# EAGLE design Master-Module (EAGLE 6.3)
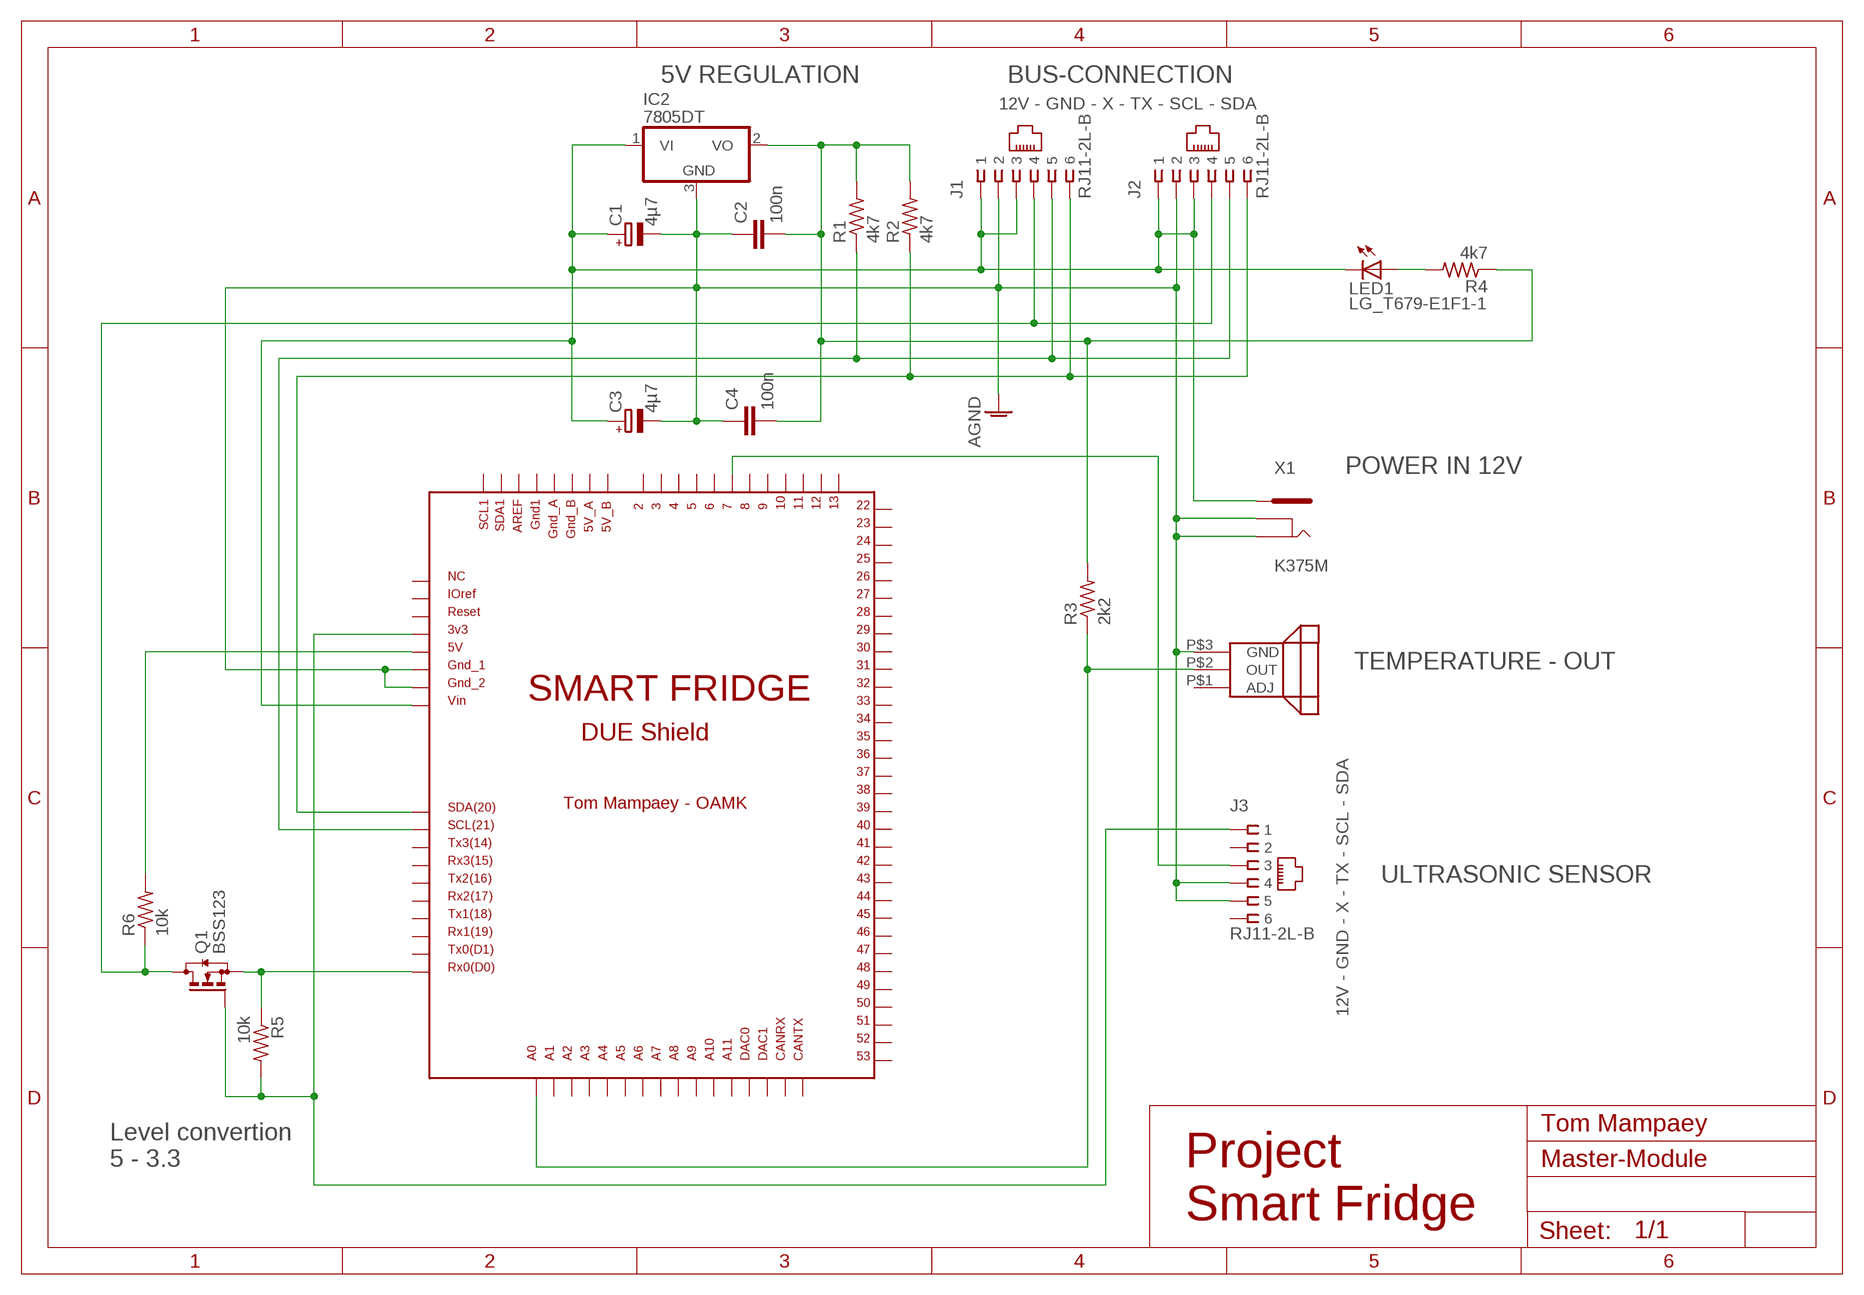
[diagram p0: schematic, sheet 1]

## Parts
C1  4µ7  CPOL-EUB  [PANASONIC_B]
C2  100n  C-EUC0603  [C0603]
C3  4µ7  CPOL-EUB  [PANASONIC_B]
C4  100n  C-EUC0603  [C0603]
IC2  7805DT  [TO252]
J1  RJ11-2L-B  [RJ11-NO_SHIELD]
J2  RJ11-2L-B  [RJ11-NO_SHIELD]
J3  RJ11-2L-B  [RJ11-NO_SHIELD]
LED1  LG_T679-E1F1-1  [PLCC2]
Q1  BSS123  [SOT23]
R1  4k7  R-US_R0402  [R0402]
R2  4k7  R-US_R0402  [R0402]
R3  2k2  R-US_R0402  [R0402]
R4  4k7  R-US_R0402  [R0402]
R5  10k  R-US_R0402  [R0402]
R6  10k  R-US_R0402  [R0402]
U$1  DUE(NORMAL)  [DUE(NORMAL)]
U$2  LM335  [LM335]
X1  K375M  [K375M]

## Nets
AGND: C1.- C2.1 C3.- C4.1 IC2.3(GND) J1.2 J2.2 J3.4 J3.5 U$1.GND_1 U$1.GND_2 U$2.P$3(GND) X1.P$1 X1.P$6
N$1: J1.6 J2.6 R2.1 U$1.SDA
N$2: J1.4 J2.4 Q1.3(D) R6.1
N$3: J1.5 J2.5 R1.1 U$1.SCL
N$4: R6.2 U$1.5V
N$5: R3.1 U$1.A0 U$2.P$2(OUT)
N$6: J3.3 U$1.7
N$7: LED1.A R4.2
N$8: C2.2 C4.2 IC2.2(VO) R1.2 R2.2 R3.2 R4.1
N$9: Q1.2(S) R5.1 U$1.RX0
N$10: C1.+ C3.+ IC2.1(VI) J1.1 J1.3 J2.1 J2.3 LED1.C U$1.VIN X1.P$7
N$14: J3.1 Q1.1(G) R5.2 U$1.3V3
Unconnected: J3.2 J3.6 U$1.2 U$1.3 U$1.4 U$1.5 U$1.5V_A U$1.5V_B U$1.6 U$1.8 U$1.9 U$1.10 U$1.11 U$1.12 U$1.13 U$1.22 U$1.23 U$1.24 U$1.25 U$1.26 U$1.27 U$1.28 U$1.29 U$1.30 U$1.31 U$1.32 U$1.33 U$1.34 U$1.35 U$1.36 U$1.37 U$1.38 U$1.39 U$1.40 U$1.41 U$1.42 U$1.43 U$1.44 U$1.45 U$1.46 U$1.47 U$1.48 U$1.49 U$1.50 U$1.51 U$1.52 U$1.53 U$1.A1 U$1.A2 U$1.A3 U$1.A4 U$1.A5 U$1.A6 U$1.A7 U$1.A8 U$1.A9 U$1.A10 U$1.A11 U$1.AREF U$1.CANRX U$1.CANTX U$1.DAC0 U$1.DAC1 U$1.GND1 U$1.GND_A U$1.GND_B U$1.IOREF U$1.NC U$1.RESET U$1.RX1 U$1.RX2 U$1.RX3 U$1.SCL1 U$1.SDA1 U$1.TX0 U$1.TX1 U$1.TX2 U$1.TX3 U$2.P$1(ADJ)

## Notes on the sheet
- 5V REGULATION | BUS-CONNECTION
- 12V - GND - X - TX - SCL - SDA
- POWER IN 12V
- TEMPERATURE - OUT
- 12V - GND - X - TX - SCL - SDA
- ULTRASONIC SENSOR
- Tom Mampaey
- Level convertion
  5 - 3.3
- Project 
  Smart Fridge

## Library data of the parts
C1 C3 = resistor:CPOL-EU: POLARIZED CAPACITOR, European symbol
C2 C4 = resistor:C-EU: CAPACITOR, European symbol
IC2 = linear:78*: Positive VOLTAGE REGULATOR Source: http://cache.national.com/ds/LM/LM78L05.pdf http://www.fairchildsemi.com/ds/LM/LM7805.pdf
J1-J3 = con-tycoelectronics:RJ11: CORCOM Modular RJ Jacks No Shield Source: www.tycoelectronics.com .. ENG_DS_1654001_1099_RJ_L_0507.pdf; MF: TYCO ELECTRONICS; MPN: RJ11-2L-B; OC_FARNELL: unknown; OC_NEWARK: 83F4463
LED1 = led:*_T679-?-1: LC TOPLED® Low Current LED; COLOR: green
Q1 = transistor-small-signal:BSS123: N-CHANNEL MOS FET
R1-R6 = rcl:R-US_: RESISTOR, American symbol
U$1 = DUE-shield custom:DUE(NORMAL)
U$2 = LM335:LM335
X1 = con-power c:K375M: K375M - DC POWER JACK 2.5mm/CENTRAL PIN Source: Data sheet

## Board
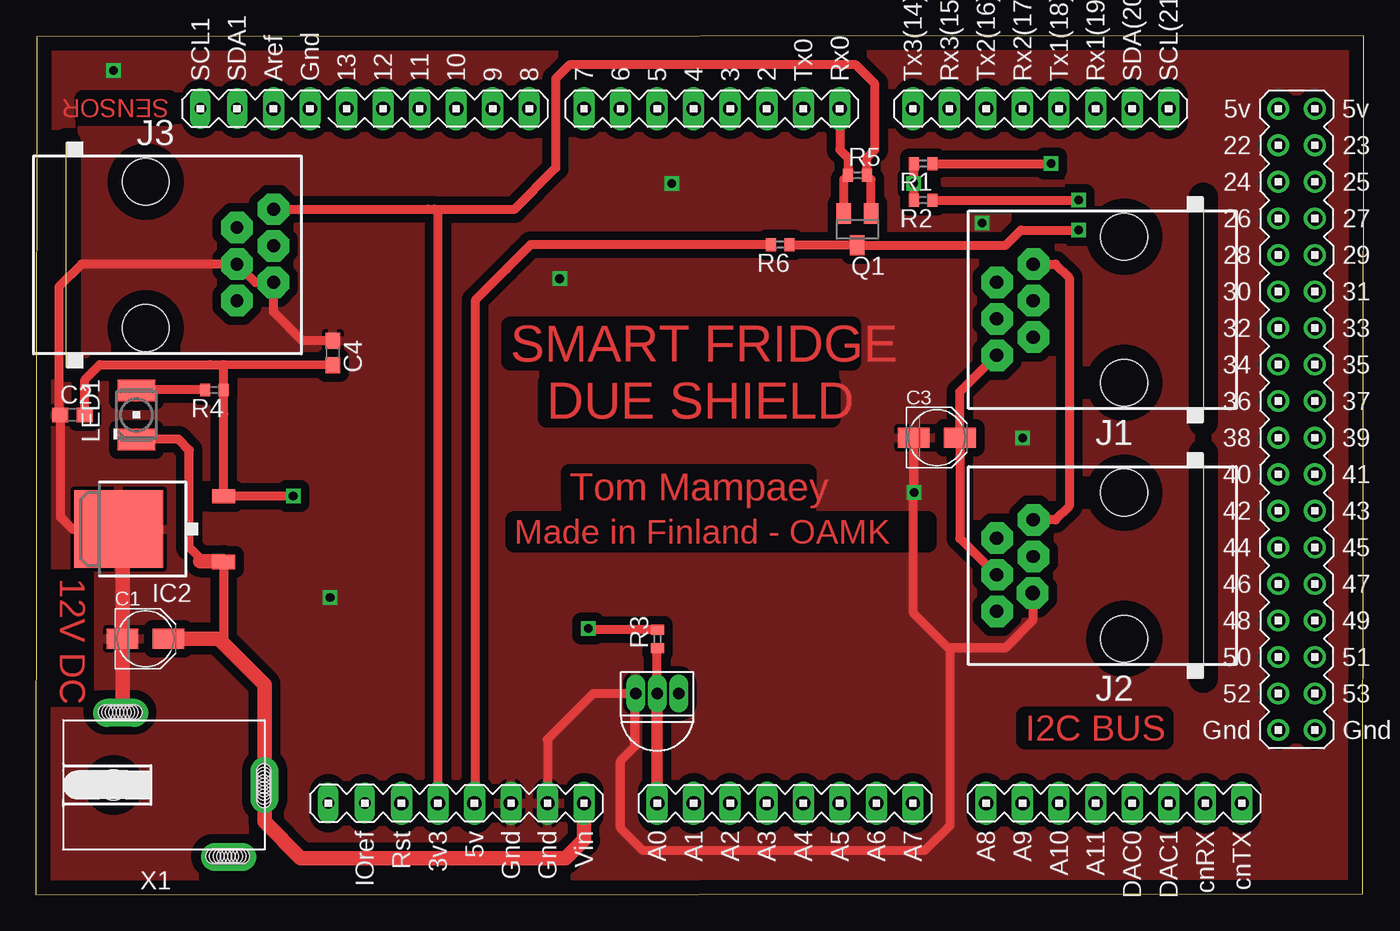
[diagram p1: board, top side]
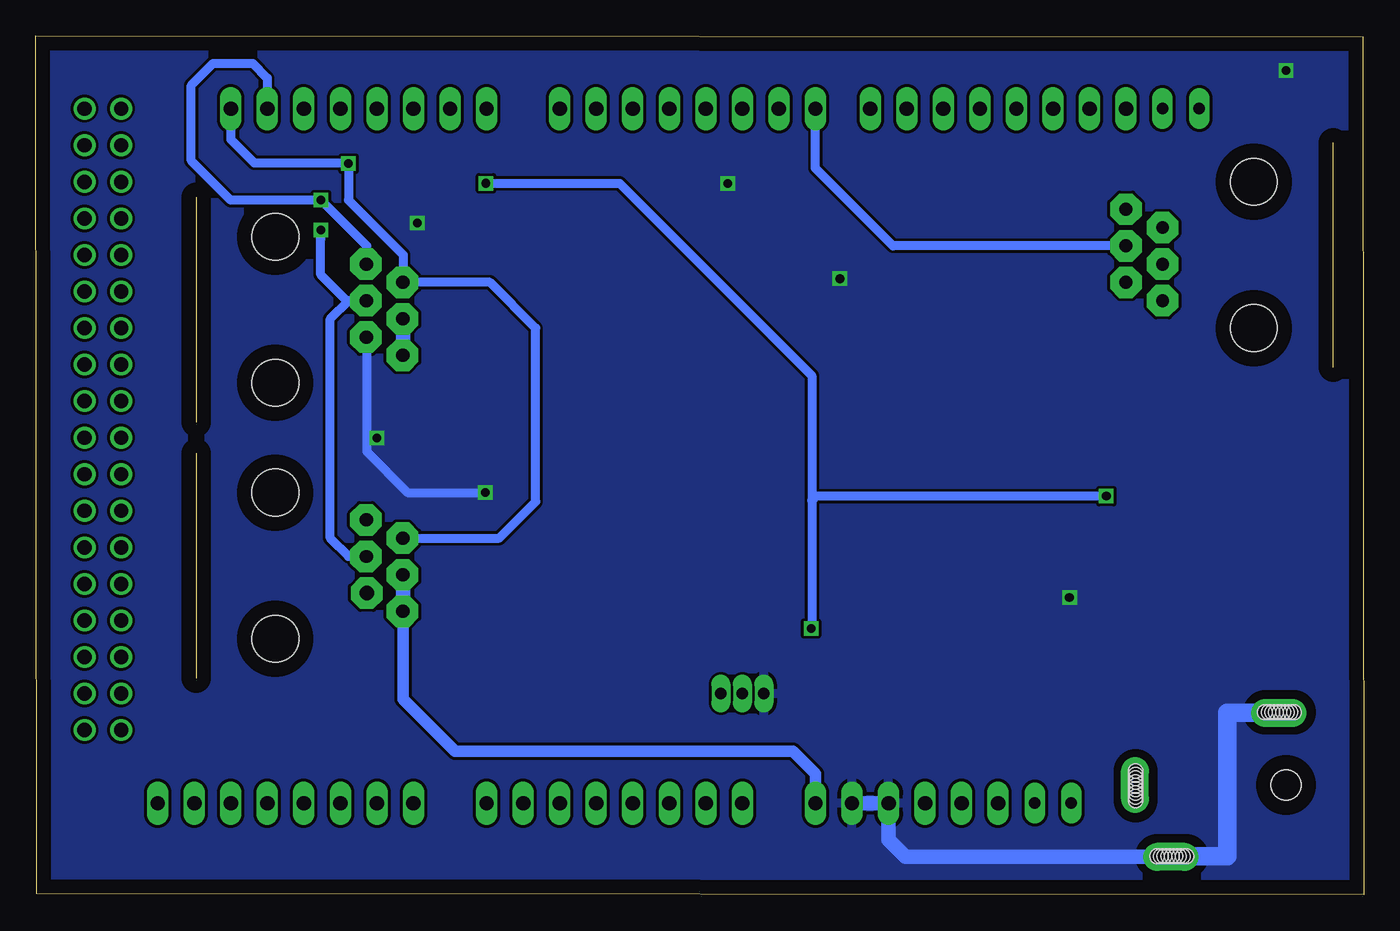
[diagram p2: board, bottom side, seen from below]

Size 92.28 x 59.66 mm. Coordinates in mm from the lower left corner, seen from the top.
Outline: 0,0 92.23,0.05 92.28,59.66 0.05,59.61 0,0
Copper layers (1*16): Top 0.035mm / dielectric 1.5mm / Bottom 0.035mm
Design rules "default": minimum track width 10mil, minimum drill 24mil, track to track 8mil, track to pad 8mil, pad to pad 8mil, via to via 8mil, smd to smd 8mil, copper to edge 40mil, drill to drill 8mil, minimum pad ring 10mil, minimum via ring 8mil, stop-mask expansion 4mil, vias tented up to drill 0mil, thermal gap 10mil

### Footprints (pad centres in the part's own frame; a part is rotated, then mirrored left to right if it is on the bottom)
PANASONIC_B = smd 2.2 x 1.4: + 1.6,0; - -1.6,0
C0603 = smd 1.1 x 1: 1 -0.85,0; 2 0.85,0
TO252 = smd 1 x 1.6: 1 -2.28,-4.8; 2 2.28,-4.8 | smd 5.4 x 6.2: 3 0,2.5
RJ11-NO_SHIELD = drill 0.9 pad 1.4: 1 -3.175,8.89; 2 -1.905,6.35; 3 -0.635,8.89; 4 0.635,6.35; 5 1.905,8.89; 6 3.175,6.35 | hole 3.251: -5.08,0; 5.08,0
PLCC2 = smd 2.6 x 1.5: A 0,1.7; C 0,-1.7
SOT23 = smd 1 x 1.4: 1 -0.95,-1.1; 2 0.95,-1.1; 3 0,1.1
R0402 = smd 0.7 x 0.9: 1 -0.65,0; 2 0.65,0
DUE(NORMAL) = drill 1 long: 2 -1.27,22.86; 3 -3.81,22.86; 3V3 -24.13,-25.4; 4 -6.35,22.86; 5 -8.89,22.86; 5V -21.59,-25.4; 6 -11.43,22.86; 7 -13.97,22.86; 8 -17.78,22.86; 9 -20.32,22.86; 10 -22.86,22.86; 11 -25.4,22.86; 12 -27.94,22.86; 13 -30.48,22.86; A0 -8.89,-25.4; A1 -6.35,-25.4; A2 -3.81,-25.4; A3 -1.27,-25.4; A4 1.27,-25.4; A5 3.81,-25.4; A6 6.35,-25.4; A7 8.89,-25.4; A8 13.97,-25.4; A9 16.51,-25.4; A10 19.05,-25.4; A11 21.59,-25.4; AREF -35.56,22.86; AREF1 -35.56,22.86; CANRX 29.21,-25.4; CANTX 31.75,-25.4; DAC0 24.13,-25.4; DAC1 26.67,-25.4; GND1 -33.02,22.86; GND_1 -19.05,-25.4; GND_2 -16.51,-25.4; RESET -26.67,-25.4; RX0 3.81,22.86; RX1 21.59,22.86; RX2 16.51,22.86; RX3 11.43,22.86; SCL 26.67,22.86; SDA 24.13,22.86; TX0 1.27,22.86; TX1 19.05,22.86; TX2 13.97,22.86; TX3 8.89,22.86; VIN -13.97,-25.4 | drill 1: 5V_A 34.29,22.86; 5V_B 36.83,22.86; 22 34.29,20.32; 23 36.83,20.32; 24 34.29,17.78; 25 36.83,17.78; 26 34.29,15.24; 27 36.83,15.24; 28 34.29,12.7; 29 36.83,12.7; 30 34.29,10.16; 31 36.83,10.16; 32 34.29,7.62; 33 36.83,7.62; 34 34.29,5.08; 35 36.83,5.08; 36 34.29,2.54; 37 36.83,2.54; 38 34.29,0; 39 36.83,0; 40 34.29,-2.54; 41 36.83,-2.54; 42 34.29,-5.08; 43 36.83,-5.08; 44 34.29,-7.62; 45 36.83,-7.62; 46 34.29,-10.16; 47 36.83,-10.16; 48 34.29,-12.7; 49 36.83,-12.7; 50 34.29,-15.24; 51 36.83,-15.24; 52 34.29,-17.78; 53 36.83,-17.78; GND_A 34.29,-20.32; GND_B 36.83,-20.32 | drill 0.8 pad 1.422 long: IOREF -29.21,-25.4; NC -31.75,-25.4; SCL1 -40.64,22.86; SDA1 -38.1,22.86
LM335 = drill 0.8 long: P$1 0,1.5; P$2 0,0; P$3 0,-1.5
K375M = drill 1 pad 1.93 long: P$1 5,3; P$6 -5,-4.5; P$7 0.004,-7.007 | hole 2.1: 0,3.5 | hole 1: -4.953,-3.429; -4.953,-3.683; -4.953,-3.937; -4.953,-4.191; -4.953,-4.445; -4.953,-4.699; -4.953,-4.953; -4.953,-5.207; -4.953,-5.461; -1.067,-6.96; -0.813,-6.96; -0.559,-6.96; -0.305,-6.96; -0.051,-6.96; 0.203,-6.96; 0.457,-6.96; 0.711,-6.96; 0.965,-6.96; 5.055,4.064; 5.055,3.81; 5.055,3.556; 5.055,3.302; 5.055,3.048; 5.055,2.794; 5.055,2.54; 5.055,2.286; 5.055,2.032

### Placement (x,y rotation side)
C1  7.62,17.78 0 top
C2  2.54,33.34 0 top
C3  62.62,31.75 0 top
C4  20.64,37.63 270 top
IC2  8.26,25.4 90 top
J1  75.64,40.64 90 top
J2  75.64,22.86 90 top
J3  7.62,44.45 270 top
LED1  6.99,33.34 0 top
Q1  57.1,46.23 180 top
R1  61.67,50.8 180 top
R2  61.67,48.26 180 top
R3  43.21,17.75 90 top
R4  12.41,35.06 180 top
R5  57.1,49.99 0 top
R6  51.74,45.16 180 top
U$1  52.07,31.75 0 top
U$2  43.18,13.97 270 top
X1  8.89,7.62 90 top

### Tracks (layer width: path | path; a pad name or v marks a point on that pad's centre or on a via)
AGND  (via drill 0.6)
  Top 0.61: U$1.GND_2 35.56,10.79 38.73,13.97 U$2.P$3 41.66,13.95 41.66,10.31 40.64,9.3 40.64,4.62 42.22,3.05 61.77,3.05 63.55,4.83 63.55,17.14 67.39,17.14 67.41,17.17 | C3.- 61.04,31.74 v61.04,27.94 61.01,27.91 61.01,19.56 63.4,17.17 67.41,17.17 | IC2.3 2.54,25.4 1.69,26.25 C2.1 1.59,33.44 1.59,42.23 3.17,43.81 J3.4 15.24,42.55 J3.5 16.51,40.49 18.52,38.48 C4.1 | J2.2 69.29,19.05 67.41,17.17
  Top 1.016: X1.P$1 6.02,12.75 C1.- 6.02,24.43 6.99,25.4 IC2.3
  Bottom 0.61: J1.2 69.29,30.8 66.43,27.94 v61.04,27.94
  Bottom 1.016: U$1.GND_2 U$1.GND_1 33.02,3.81 31.83,2.62 X1.P$6 13.31,2.54
  Bottom 1.27: X1.P$1 9.47,12.62 9.47,2.67 13.39,2.67 X1.P$6
  other vias: 20.45,20.65 5.38,57.28 44.2,49.4 68.58,31.72 36.4,42.8 65.76,46.66
  pour Bottom: 0.05,59.61 92.23,59.61 92.23,0.05 0.05,0.05
  pour Top (isolate 0.61): 0.05,59.61 92.23,59.61 92.23,0.05 0.03,0.05 0.03,59.61
N$1  (via drill 0.6)
  Top 0.61: R2.1 v72.47,48.26 | J1.6 70.88,43.81 71.83,42.86 71.83,26.99 70.88,26.04 J2.6
  Bottom 0.61: J1.6 69.29,45.09 v72.47,48.26 78.74,48.26 81.48,51 81.48,56.24 79.96,57.76 77.22,57.76 76.2,56.74 U$1.SDA
N$2  (via drill 0.6)
  Top 0.61: v72.47,46.18 68.48,46.18 67.43,45.13 Q1.3 52.56,45.13 R6.1
  Bottom 0.61: J2.4 70.56,23.5 71.83,24.77 71.83,40.01 70.56,41.27 | J1.4 70.56,41.27 | 70.56,41.27 70.69,41.27 72.49,43.08 72.49,45.54 v72.47,46.18
N$3  (via drill 0.6)
  Top 0.61: R1.1 v70.56,50.8
  Bottom 0.61: J2.5 60.08,24.77 57.54,27.3 57.54,39.37 60.72,42.55 J1.5 66.75,44.45 70.56,48.26 v70.56,50.8 70.61,50.85 77.11,50.85 78.74,52.48 U$1.SCL
N$4
  Top 0.61: U$1.5V 30.53,6.4 30.53,41.3 32.72,43.48 33.66,44.44 34.39,45.16 R6.2
N$5
  Top 0.61: U$2.P$2 43.18,17.08 R3.1
  Top 0.813: U$1.A0 U$2.P$2
N$6
  Bottom 0.61: J3.3 32.7,45.09 38.1,50.48 U$1.7
N$7
  Top 0.61: R4.2 7.01,35.06 LED1.A
N$8  (via drill 0.6)
  Top 0.61: C2.2 3.39,35.77 4.45,36.83 13.03,36.83 | 13.03,36.83 13.02,35.88 13.02,34.94 R4.1 13.05,33.39 IC2.2 v17.88,27.69 | C4.2 12.12,36.83 13.03,36.83 | R1.2 R2.2 61.02,49.42 60.96,49.48 61.01,49.58 v61.01,49.43 | 38.48,18.41 v38.41,18.49 38.49,18.41 R3.2
  Bottom 0.61: v61.01,49.43 51.71,49.43 38.35,36.07 38.35,27.38 | 38.35,27.38 38.35,18.54 v38.41,18.49 | v17.88,27.69 38.05,27.69 38.35,27.38
N$9
  Top 0.61: Q1.2 56.15,49.69 R5.1 56.44,51.21 55.88,51.77 U$1.RX0
N$10
  Top 0.61: J2.3 64.22,24.75 C3.+ 64.22,34.94 J1.1 | IC2.1 13.05,17.63 12.95,17.53 | 11.43,23.18 11.43,23.37 10.67,24.13 10.67,30.89 9.91,31.65 LED1.C
  Top 1.016: U$1.VIN 38.1,3.81 36.83,2.54 18.41,2.54 15.9,5.06 X1.P$7 15.9,14.58 12.95,17.53 12.7,17.78 C1.+ | 11.43,23.18 13,23.18 IC2.1
  Bottom 0.813: U$1.VIN 38.1,8.38 39.67,9.96 63.14,9.96 66.75,13.56 J2.1
  Bottom 1.016: J1.1 J1.3 | J2.1 J2.3
N$12  (via drill 0.9 pad 2.18)
  other vias: 13.97,46.35
N$13  (via drill 0.9 pad 2.18)
  other vias: 16.51,45.09
N$14  (via drill 0.9 pad 2.18)
  Top 0.61: J3.1 27.28,47.62 | 27.28,47.62 27.69,47.62 27.94,47.37 U$1.3V3 | Q1.1 58.05,49.69 R5.2 57.75,51.2 58.32,51.77 58.32,56.34 57,57.66 37.08,57.66 36.12,56.69 36.12,50.49 33.22,47.6 27.3,47.6 27.28,47.62
  other vias: 16.51,47.62
N$15  (via drill 0.9 pad 2.18)
  other vias: 13.97,43.81
N$16  (via drill 0.9 pad 2.18)
  other vias: 16.51,42.55
N$17  (via drill 0.9 pad 2.18)
  other vias: 13.97,41.27
N$18  (via drill 0.9 pad 2.18)
  other vias: 69.34,43.81
N$19  (via drill 0.9 pad 2.18)
  other vias: 66.8,42.55
N$20  (via drill 0.9 pad 2.18)
  other vias: 69.34,41.27
N$21  (via drill 0.9 pad 2.18)
  other vias: 66.8,40.01
N$22  (via drill 0.9 pad 2.18)
  other vias: 66.8,37.47
N$23  (via drill 0.9 pad 2.18)
  other vias: 69.34,26.04
N$24  (via drill 0.9 pad 2.18)
  other vias: 69.34,23.5
N$25  (via drill 0.9 pad 2.18)
  other vias: 66.8,22.23
N$26  (via drill 0.9 pad 2.18)
  other vias: 66.8,19.68
N$27  (via drill 0.9 pad 2.18)
  other vias: 69.34,38.73
N$28  (via drill 0.9 pad 2.18)
  other vias: 66.8,24.77
N$29  (via drill 1 pad 2.18)
  other vias: 69.29,20.95

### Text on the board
Top: SENSOR | SMART FRIDGE | DUE SHIELD | Tom Mampaey | Made in Finland - OAMK | 12V DC | I2C BUS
